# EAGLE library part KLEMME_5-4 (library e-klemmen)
Klemme 5 4
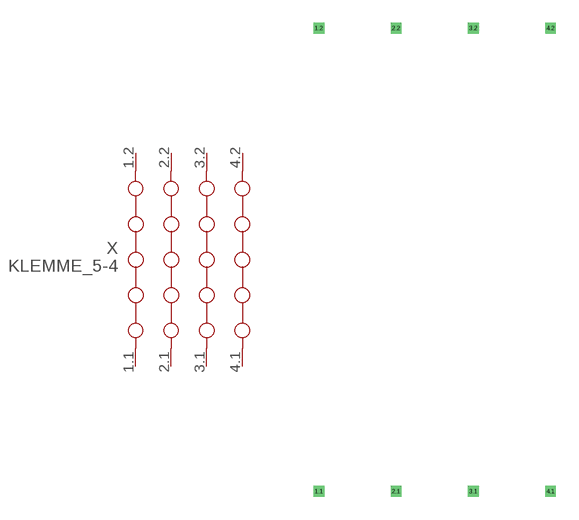
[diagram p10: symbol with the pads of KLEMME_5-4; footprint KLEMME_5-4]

Designator prefix X

## KLEMME_5-4  [KLEMME_5-4]
1.1  1.1  pas
1.2  1.2  pas
2.1  2.1  pas
2.2  2.2  pas
3.1  3.1  pas
3.2  3.2  pas
4.1  4.1  pas
4.2  4.2  pas

## Footprint KLEMME_5-4 (pad centres in mm)
Dummy
drill 0.2 pad 0.6 square: 1.1 0,-15.24; 1.2 0,15.24; 2.1 5.08,-15.24; 2.2 5.08,15.24; 3.1 10.16,-15.24; 3.2 10.16,15.24; 4.1 15.24,-15.24; 4.2 15.24,15.24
